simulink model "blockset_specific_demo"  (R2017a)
settings: Solver=ode45  StartTime=0.0  StopTime=2  RelTol=1e-3  EnableMultiTasking=on
InitFcn:
  | VoutDC_Matlab = 300;
  | 
  | % Load profile
  | Ploadprofile_max = 1000;
  | Imax = Ploadprofile_max/VoutDC_Matlab;
  | 
  | % Resistive load
  | Presisitve = 1000;
  | Pmax = Ploadprofile_max + Presisitve;
undefined symbols (not defined in the file): plecs, slselsubs
libraries: simulink x1, plecslib_extras2 x1

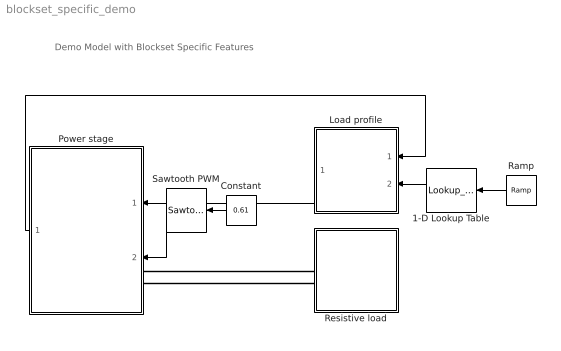
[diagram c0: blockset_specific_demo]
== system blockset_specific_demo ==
  note: Demo Model with Blockset Specific Features
  1-D Lookup Table : Lookup_n-D  NumberOfTableDimensions=1  BreakpointsForDimension1=[0 0.5 1 1.5 1.501 2]  BreakpointsForDimension5=slselsubs({[1:3], [1:3], [1:3], [1:3], [1:3], [1:3], [1:3], [1:3], [1:3], [1:3], [1:3], [1:3], [1:3], [1:3], [1:3], [1:3], [1:3], [1:3], [1:3], [1:3], [1:3], [1:3], [1:3], [1:3], [1:3], [1:3]}, 1)  BreakpointsForDimension6=slselsubs({[1:3], [1:3], [1:3], [1:3], [1:3], [1:3], [1:3], [1:3], [1:3], [1:3], [1:3], [1:3], [1:3], [1:3], [1:3], [1:3], [1:3], [1:3], [1:3], [1:3], [1:3], [1:3], [1:3], [1:3], [1:3], [1:3]}, 2)  BreakpointsForDimension7=slselsubs({[1:3], [1:3], [1:3], [1:3], [1:3], [1:3], [1:3], [1:3], [1:3], [1:3], [1:3], [1:3], [1:3], [1:3], [1:3], [1:3], [1:3], [1:3], [1:3], [1:3], [1:3], [1:3], [1:3], [1:3], [1:3], [1:3]}, 3)  BreakpointsForDimension8=slselsubs({[1:3], [1:3], [1:3], [1:3], [1:3], [1:3], [1:3], [1:3], [1:3], [1:3], [1:3], [1:3], [1:3], [1:3], [1:3], [1:3], [1:3], [1:3], [1:3], [1:3], [1:3], [1:3], [1:3], [1:3], [1:3], [1:3]}, 4)  BreakpointsForDimension9=slselsubs({[1:3], [1:3], [1:3], [1:3], [1:3], [1:3], [1:3], [1:3], [1:3], [1:3], [1:3], [1:3], [1:3], [1:3], [1:3], [1:3], [1:3], [1:3], [1:3], [1:3], [1:3], [1:3], [1:3], [1:3], [1:3], [1:3]}, 5)  BreakpointsForDimension10=slselsubs({[1:3], [1:3], [1:3], [1:3], [1:3], [1:3], [1:3], [1:3], [1:3], [1:3], [1:3], [1:3], [1:3], [1:3], [1:3], [1:3], [1:3], [1:3], [1:3], [1:3], [1:3], [1:3], [1:3], [1:3], [1:3], [1:3]}, 6)  BreakpointsForDimension11=slselsubs({[1:3], [1:3], [1:3], [1:3], [1:3], [1:3], [1:3], [1:3], [1:3], [1:3], [1:3], [1:3], [1:3], [1:3], [1:3], [1:3], [1:3], [1:3], [1:3], [1:3], [1:3], [1:3], [1:3], [1:3], [1:3], [1:3]}, 7)  BreakpointsForDimension12=slselsubs({[1:3], [1:3], [1:3], [1:3], [1:3], [1:3], [1:3], [1:3], [1:3], [1:3], [1:3], [1:3], [1:3], [1:3], [1:3], [1:3], [1:3], [1:3], [1:3], [1:3], [1:3], [1:3], [1:3], [1:3], [1:3], [1:3]}, 8)  BreakpointsForDimension13=slselsubs({[1:3], [1:3], [1:3], [1:3], [1:3], [1:3], [1:3], [1:3], [1:3], [1:3], [1:3], [1:3], [1:3], [1:3], [1:3], [1:3], [1:3], [1:3], [1:3], [1:3], [1:3], [1:3], [1:3], [1:3], [1:3], [1:3]}, 9)  BreakpointsForDimension14=slselsubs({[1:3], [1:3], [1:3], [1:3], [1:3], [1:3], [1:3], [1:3], [1:3], [1:3], [1:3], [1:3], [1:3], [1:3], [1:3], [1:3], [1:3], [1:3], [1:3], [1:3], [1:3], [1:3], [1:3], [1:3], [1:3], [1:3]}, 10)  BreakpointsForDimension15=slselsubs({[1:3], [1:3], [1:3], [1:3], [1:3], [1:3], [1:3], [1:3], [1:3], [1:3], [1:3], [1:3], [1:3], [1:3], [1:3], [1:3], [1:3], [1:3], [1:3], [1:3], [1:3], [1:3], [1:3], [1:3], [1:3], [1:3]}, 11)  BreakpointsForDimension16=slselsubs({[1:3], [1:3], [1:3], [1:3], [1:3], [1:3], [1:3], [1:3], [1:3], [1:3], [1:3], [1:3], [1:3], [1:3], [1:3], [1:3], [1:3], [1:3], [1:3], [1:3], [1:3], [1:3], [1:3], [1:3], [1:3], [1:3]}, 12)  BreakpointsForDimension17=slselsubs({[1:3], [1:3], [1:3], [1:3], [1:3], [1:3], [1:3], [1:3], [1:3], [1:3], [1:3], [1:3], [1:3], [1:3], [1:3], [1:3], [1:3], [1:3], [1:3], [1:3], [1:3], [1:3], [1:3], [1:3], [1:3], [1:3]}, 13)  BreakpointsForDimension18=slselsubs({[1:3], [1:3], [1:3], [1:3], [1:3], [1:3], [1:3], [1:3], [1:3], [1:3], [1:3], [1:3], [1:3], [1:3], [1:3], [1:3], [1:3], [1:3], [1:3], [1:3], [1:3], [1:3], [1:3], [1:3], [1:3], [1:3]}, 14)  BreakpointsForDimension19=slselsubs({[1:3], [1:3], [1:3], [1:3], [1:3], [1:3], [1:3], [1:3], [1:3], [1:3], [1:3], [1:3], [1:3], [1:3], [1:3], [1:3], [1:3], [1:3], [1:3], [1:3], [1:3], [1:3], [1:3], [1:3], [1:3], [1:3]}, 15)  BreakpointsForDimension20=slselsubs({[1:3], [1:3], [1:3], [1:3], [1:3], [1:3], [1:3], [1:3], [1:3], [1:3], [1:3], [1:3], [1:3], [1:3], [1:3], [1:3], [1:3], [1:3], [1:3], [1:3], [1:3], [1:3], [1:3], [1:3], [1:3], [1:3]}, 16)  BreakpointsForDimension21=slselsubs({[1:3], [1:3], [1:3], [1:3], [1:3], [1:3], [1:3], [1:3], [1:3], [1:3], [1:3], [1:3], [1:3], [1:3], [1:3], [1:3], [1:3], [1:3], [1:3], [1:3], [1:3], [1:3], [1:3], [1:3], [1:3], [1:3]}, 17)  BreakpointsForDimension22=slselsubs({[1:3], [1:3], [1:3], [1:3], [1:3], [1:3], [1:3], [1:3], [1:3], [1:3], [1:3], [1:3], [1:3], [1:3], [1:3], [1:3], [1:3], [1:3], [1:3], [1:3], [1:3], [1:3], [1:3], [1:3], [1:3], [1:3]}, 18)  BreakpointsForDimension23=slselsubs({[1:3], [1:3], [1:3], [1:3], [1:3], [1:3], [1:3], [1:3], [1:3], [1:3], [1:3], [1:3], [1:3], [1:3], [1:3], [1:3], [1:3], [1:3], [1:3], [1:3], [1:3], [1:3], [1:3], [1:3], [1:3], [1:3]}, 19)  BreakpointsForDimension24=slselsubs({[1:3], [1:3], [1:3], [1:3], [1:3], [1:3], [1:3], [1:3], [1:3], [1:3], [1:3], [1:3], [1:3], [1:3], [1:3], [1:3], [1:3], [1:3], [1:3], [1:3], [1:3], [1:3], [1:3], [1:3], [1:3], [1:3]}, 20)  BreakpointsForDimension25=slselsubs({[1:3], [1:3], [1:3], [1:3], [1:3], [1:3], [1:3], [1:3], [1:3], [1:3], [1:3], [1:3], [1:3], [1:3], [1:3], [1:3], [1:3], [1:3], [1:3], [1:3], [1:3], [1:3], [1:3], [1:3], [1:3], [1:3]}, 21)  BreakpointsForDimension26=slselsubs({[1:3], [1:3], [1:3], [1:3], [1:3], [1:3], [1:3], [1:3], [1:3], [1:3], [1:3], [1:3], [1:3], [1:3], [1:3], [1:3], [1:3], [1:3], [1:3], [1:3], [1:3], [1:3], [1:3], [1:3], [1:3], [1:3]}, 22)  BreakpointsForDimension27=slselsubs({[1:3], [1:3], [1:3], [1:3], [1:3], [1:3], [1:3], [1:3], [1:3], [1:3], [1:3], [1:3], [1:3], [1:3], [1:3], [1:3], [1:3], [1:3], [1:3], [1:3], [1:3], [1:3], [1:3], [1:3], [1:3], [1:3]}, 23)  BreakpointsForDimension28=slselsubs({[1:3], [1:3], [1:3], [1:3], [1:3], [1:3], [1:3], [1:3], [1:3], [1:3], [1:3], [1:3], [1:3], [1:3], [1:3], [1:3], [1:3], [1:3], [1:3], [1:3], [1:3], [1:3], [1:3], [1:3], [1:3], [1:3]}, 24)  BreakpointsForDimension29=slselsubs({[1:3], [1:3], [1:3], [1:3], [1:3], [1:3], [1:3], [1:3], [1:3], [1:3], [1:3], [1:3], [1:3], [1:3], [1:3], [1:3], [1:3], [1:3], [1:3], [1:3], [1:3], [1:3], [1:3], [1:3], [1:3], [1:3]}, 25)  BreakpointsForDimension30=slselsubs({[1:3], [1:3], [1:3], [1:3], [1:3], [1:3], [1:3], [1:3], [1:3], [1:3], [1:3], [1:3], [1:3], [1:3], [1:3], [1:3], [1:3], [1:3], [1:3], [1:3], [1:3], [1:3], [1:3], [1:3], [1:3], [1:3]}, 26)  Table=[0 0 Imax Imax 0 0]  RndMeth=Simplest
  Constant : Constant  Value=0.61
  Load profile : Subsystem  LoadFcn=plecs('sl', 200);  InitFcn=plecs('sl', 214);  StartFcn=plecs('sl', 208);  StopFcn=plecs('sl', 209);  ClipboardFcn=plecs('sl', 212, 78);
  Power stage : Subsystem  LoadFcn=plecs('sl', 200);  InitFcn=plecs('sl', 214);  StartFcn=plecs('sl', 208);  StopFcn=plecs('sl', 209);  ClipboardFcn=plecs('sl', 212, 77);
  Ramp : simulink/Sources/Ramp  slope=1  start=0  X0=0
  Resistive load : Subsystem  LoadFcn=plecs('sl', 200);  InitFcn=plecs('sl', 214);  StartFcn=plecs('sl', 208);  StopFcn=plecs('sl', 209);  ClipboardFcn=plecs('sl', 212, 76);
  Sawtooth PWM : plecslib_extras2/Modulators/Sawtooth PWM  sampling=regular  ramp=falling  fc=10e3  offset=0  input_limits=[0 1]  output_values=[0 1]
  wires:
  Load profile/1(Iout) -> Power stage/1(Iin)
  Ramp/1 -> 1-D Lookup Table/1
  1-D Lookup Table/1 -> Load profile/2(Load profile)
  Power stage/1(Vout) -> Load profile/1(Vin)
  Constant/1 -> Sawtooth PWM/1
  Sawtooth PWM/1 -> Power stage/2(PWM)
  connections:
  Resistive load/LConn1 -- Power stage/LConn1
  Power stage/LConn2 -- Resistive load/LConn2

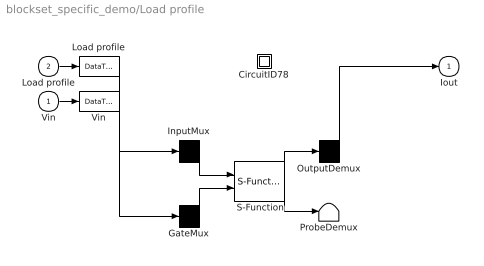
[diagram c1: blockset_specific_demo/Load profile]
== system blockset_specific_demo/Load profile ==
  Vin : Inport  PortDimensions=1
  Load profile : Inport  Port=2  PortDimensions=1
  " CircuitID78 " : Subsystem
  " GateMux " : Mux  Inputs=[ 1 ]
  " InputMux " : Mux  Inputs=[ 1 ]
  " Load profile " : DataTypeConversion
  " OutputDemux " : Demux  Outputs=[ 1 ]
  " ProbeDemux " : Terminator
  " S-Function " : S-Function  FunctionName=plecs  SFunctionDeploymentMode=off  EnableBusSupport=off
  " Vin " : DataTypeConversion
  Iout : Outport  PortDimensions=1
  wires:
  " InputMux "/1 -> " S-Function "/1
  " GateMux "/1 -> " S-Function "/2
  " S-Function "/1 -> " OutputDemux "/1
  " S-Function "/2 -> " ProbeDemux "/1
  Load profile/1 -> " Load profile "/1
  " Load profile "/1 -> " InputMux "/1
  Vin/1 -> " Vin "/1
  " Vin "/1 -> " GateMux "/1
  " OutputDemux "/1 -> Iout/1

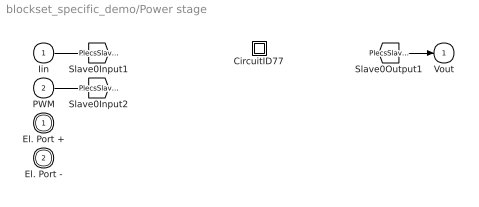
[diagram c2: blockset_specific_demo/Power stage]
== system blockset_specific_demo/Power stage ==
  Iin : Inport  PortDimensions=1
  PWM : Inport  Port=2  PortDimensions=1
  " CircuitID77 " : Subsystem
  El. Port + : PMIOPort  Side=Left
  El. Port - : PMIOPort  Port=2  Side=Left
  Vout : Outport  PortDimensions=1
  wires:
  Iin/1 -> [PlecsSlave0Input1]
  [PlecsSlave0Output1] -> Vout/1
  PWM/1 -> [PlecsSlave0Input2]

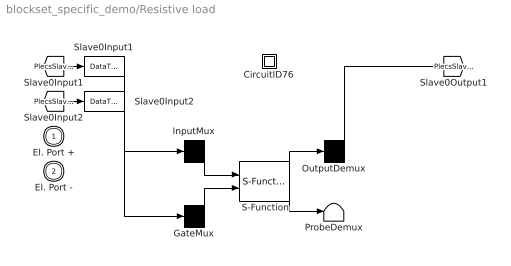
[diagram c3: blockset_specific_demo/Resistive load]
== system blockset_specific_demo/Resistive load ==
  "  Slave0Input1  " : DataTypeConversion
  "  Slave0Input2  " : DataTypeConversion
  " CircuitID76 " : Subsystem
  " GateMux " : Mux  Inputs=[ 1 ]
  " InputMux " : Mux  Inputs=[ 1 ]
  " OutputDemux " : Demux  Outputs=[ 1 ]
  " ProbeDemux " : Terminator
  " S-Function " : S-Function  FunctionName=plecs  SFunctionDeploymentMode=off  EnableBusSupport=off
  El. Port + : PMIOPort  Side=Left
  El. Port - : PMIOPort  Port=2  Side=Left
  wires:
  " InputMux "/1 -> " S-Function "/1
  " GateMux "/1 -> " S-Function "/2
  " S-Function "/1 -> " OutputDemux "/1
  " S-Function "/2 -> " ProbeDemux "/1
  [PlecsSlave0Input1] -> "  Slave0Input1  "/1
  "  Slave0Input1  "/1 -> " InputMux "/1
  [PlecsSlave0Input2] -> "  Slave0Input2  "/1
  "  Slave0Input2  "/1 -> " GateMux "/1
  " OutputDemux "/1 -> [PlecsSlave0Output1]

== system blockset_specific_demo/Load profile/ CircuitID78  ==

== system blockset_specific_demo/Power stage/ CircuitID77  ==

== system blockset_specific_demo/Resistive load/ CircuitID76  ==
